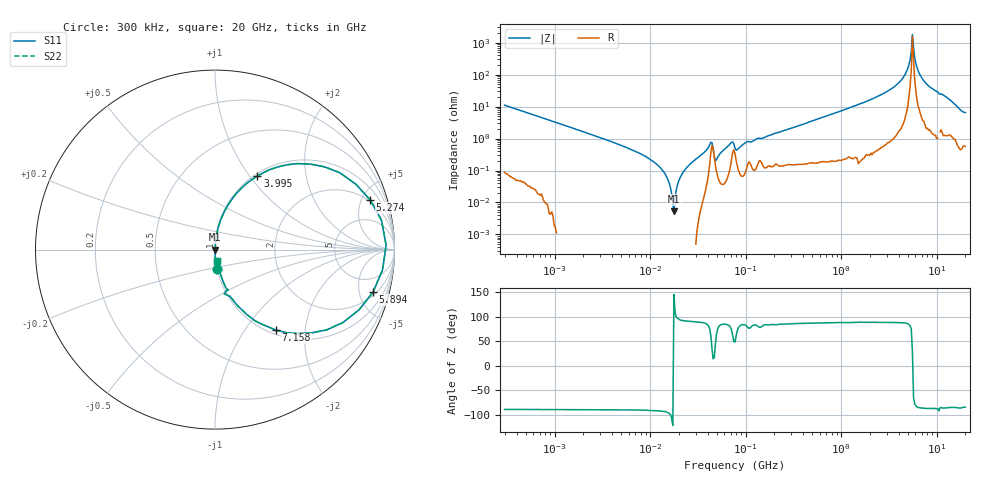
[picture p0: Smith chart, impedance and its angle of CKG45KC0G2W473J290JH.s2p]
! S-Parameter Data Generated by TDK Corporation
! Copyright(C) 2022 TDK Corporation.
! All Rights Reserved.
! TDK P/N: CKG45KC0G2W473J290JH (Multilayer Ceramic Chip Capacitor)
! Property: C=47nF
! Size(LxWxT): 5x3.5x2.9mm
! Model Type: s2p (Touchstone File Format Version 1.0)
! Frequency: DC=Yes Start=0.3MHz Stop=20000MHz 402points Log-sweep
! Model Generated on Apr. 15, 2022
! Port Assignments:
!  1 ---| |--- 2
! Applicable Conditions:
!  Temperature = 25 degC
!  DC Bias Voltage = 0 V
!  Small Signal Operation
! Terms and conditions regarding TDK Simulation Models
! (1)This simulation model is being provided solely for informational purposes. Please refer to the specifications of the products in terms of detailed characteristics of such products.
! (2)In no event shall TDK Corporation of any of its subsidiaries be liable for any loss or damage arising, directly or indirectly,
!  From any information contained in this simulation model, including, but not limited to loss or damages arising from any inaccuracies, omissions or errors in connection with such information.
! (3)Any and all copyrights on this simulation model are owned by TDK Corporation.
!  Duplication or redistribution of this simulation model without prior written permission from TDK Corporation is prohibited.
! (4)This simulation model is subject to any modification or change without any prior notice.
! (5)Neither TDK Corporation nor any of its subsidiaries shall make any warranty, express or implied,
!  Including but not limited to the correctness, implied warranties of merchantability and fitness for a particular purpose with respect to this simulation models.
! (6)The use of this simulation model shall be deemed to have consented to the terms and conditions hereof.
# Hz S MA R 50
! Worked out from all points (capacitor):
!   401 points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, 300 kHz to 20 GHz, reference 50 ohm
!   read as one part in series: C = 48 nF near 317.1 kHz
!   lowest |Z| = 5.31 mohm at 17.78 MHz (marker M1)
!   series resonance near 17.64 MHz, so ESL is about 1.7 nH
!   S11 on the Smith chart (normalised r, x): 300 kHz: 1.00, -0.22; 3.995 GHz: 1.03, +1.09; 5.274 GHz: 1.85, +5.82; 5.894 GHz: 2.41, -6.76; 7.158 GHz: 1.07, -1.41; 20 GHz: 1.01, -0.13
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300000  0.1097 -83.2  0.9931 6.3  0.9931 6.3  0.1097 -83.2
1928084  0.01694 -89.2  0.9999 1.0  0.9999 1.0  0.01694 -89.2
7111075  0.003911 -90.5  1 0.2  1 0.2  0.003911 -90.5
1.239169e7  0.001351 -92.5  1 0.1  1 0.1  0.001351 -92.5
1.505044e7  0.0005983 -95.4  1 0.0  1 0.0  0.0005983 -95.4
1.777902e7  5.307e-05 145.8  1 -0.0  1 -0.0  5.307e-05 145.8
2.282683e7  0.0009938 92.0  1 -0.1  1 -0.1  0.0009938 92.0
4.204948e7  0.006293 75.4  0.9984 -0.3  0.9984 -0.3  0.006293 75.4
4.967287e7  0.002204 65.8  0.9991 -0.1  0.9991 -0.1  0.002204 65.8
6.931649e7  0.006927 78.6  0.9987 -0.4  0.9987 -0.4  0.006927 78.6
7.964076e7  0.004311 61.0  0.9979 -0.2  0.9979 -0.2  0.004311 61.0
4.978292e8  0.03551 85.2  0.9976 -2.0  0.9976 -2.0  0.03551 85.2
3.199522e9  0.3095 70.7  0.9438 -18.0  0.9438 -18.0  0.3095 70.7
3.995427e9  0.4733 60.0  0.8668 -28.2  0.8668 -28.2  0.4733 60.0
4.85268e9  0.7653 37.1  0.6036 -49.8  0.6036 -49.8  0.7653 37.1
5.274253e9  0.9075 17.8  0.3087 -63.9  0.3087 -63.9  0.9075 17.8
5.575457e9  0.9537 1.5  0.053 -28.4  0.053 -28.4  0.9537 1.5
5.893863e9  0.9121 -15.0  0.2641 63.2  0.2641 63.2  0.9121 -15.0
6.405888e9  0.7659 -35.7  0.586 49.8  0.586 49.8  0.7659 -35.7
7.158441e9  0.5637 -52.8  0.7973 34.3  0.7973 34.3  0.5637 -52.8
9.989315e9  0.2831 -71.6  0.9496 16.4  0.9496 16.4  0.2831 -71.6
2e10  0.06391 -81.2  0.9923 3.6  0.9923 3.6  0.06391 -81.2
